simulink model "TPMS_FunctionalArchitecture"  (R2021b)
settings: Solver=VariableStepAuto  StartTime=0.0  StopTime=10.0  RelTol=1e-3

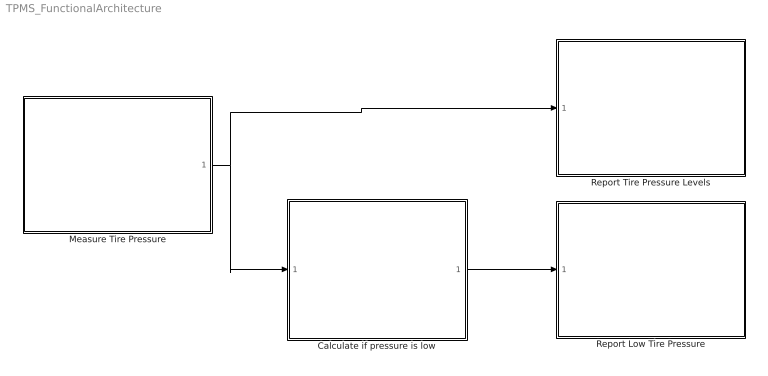
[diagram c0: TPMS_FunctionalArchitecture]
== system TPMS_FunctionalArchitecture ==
  Calculate if pressure is low : Subsystem
  Measure Tire Pressure : Subsystem
  Report Low Tire Pressure : Subsystem
  Report Tire Pressure Levels : Subsystem
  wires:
  Calculate if pressure is low/1(Bus Element Out1) -> Report Low Tire Pressure/1(Bus Element In1)
  Measure Tire Pressure/1(Bus Element Out1) -> Report Tire Pressure Levels/1(Bus Element In1), Calculate if pressure is low/1(Bus Element In1)

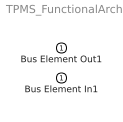
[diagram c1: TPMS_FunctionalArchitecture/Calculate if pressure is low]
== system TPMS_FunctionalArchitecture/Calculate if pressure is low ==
  Bus Element In1 : Inport
  Bus Element Out1 : Outport

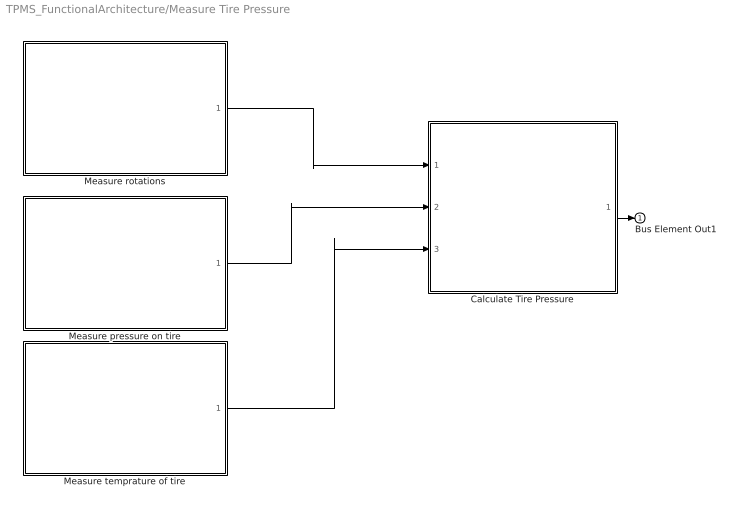
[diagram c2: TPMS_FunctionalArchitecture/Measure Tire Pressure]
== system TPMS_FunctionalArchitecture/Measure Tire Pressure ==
  Calculate Tire Pressure : Subsystem
  Measure pressure on tire : Subsystem
  Measure rotations : Subsystem
  Measure temprature of tire : Subsystem
  Bus Element Out1 : Outport
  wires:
  Measure temprature of tire/1(Bus Element Out1) -> Calculate Tire Pressure/3(Bus Element In1)
  Measure pressure on tire/1(Bus Element Out1) -> Calculate Tire Pressure/2(Bus Element In2)
  Measure rotations/1(Bus Element Out1) -> Calculate Tire Pressure/1(Bus Element In3)
  Calculate Tire Pressure/1(Bus Element Out1) -> Bus Element Out1/1

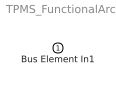
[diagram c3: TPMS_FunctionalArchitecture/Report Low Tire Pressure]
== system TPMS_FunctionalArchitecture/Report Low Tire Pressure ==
  Bus Element In1 : Inport

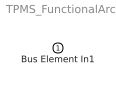
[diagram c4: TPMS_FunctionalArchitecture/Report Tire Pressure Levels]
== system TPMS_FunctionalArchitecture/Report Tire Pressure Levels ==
  Bus Element In1 : Inport

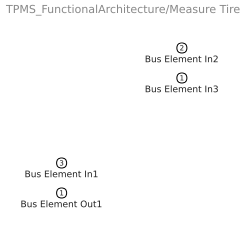
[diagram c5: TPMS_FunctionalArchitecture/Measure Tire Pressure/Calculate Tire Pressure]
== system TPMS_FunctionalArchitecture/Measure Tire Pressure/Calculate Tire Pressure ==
  Bus Element In3 : Inport
  Bus Element In2 : Inport  Port=2
  Bus Element In1 : Inport  Port=3
  Bus Element Out1 : Outport

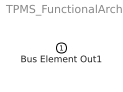
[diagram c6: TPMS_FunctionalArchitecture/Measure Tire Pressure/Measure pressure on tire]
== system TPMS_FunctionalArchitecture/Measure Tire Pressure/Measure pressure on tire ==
  Bus Element Out1 : Outport

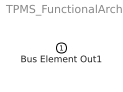
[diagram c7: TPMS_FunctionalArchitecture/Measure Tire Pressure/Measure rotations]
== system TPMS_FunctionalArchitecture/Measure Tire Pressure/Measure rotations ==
  Bus Element Out1 : Outport

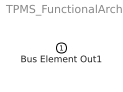
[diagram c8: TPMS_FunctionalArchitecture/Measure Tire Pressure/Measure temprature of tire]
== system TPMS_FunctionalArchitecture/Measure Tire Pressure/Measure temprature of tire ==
  Bus Element Out1 : Outport
